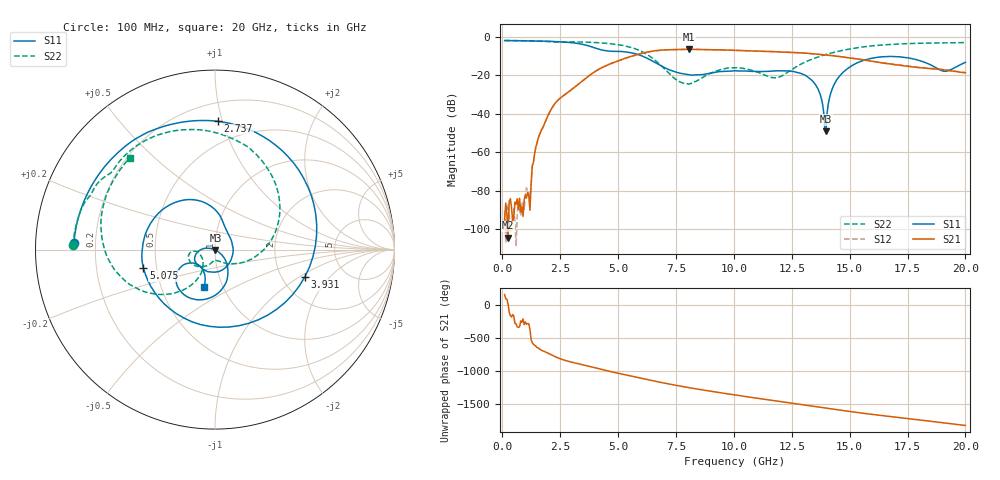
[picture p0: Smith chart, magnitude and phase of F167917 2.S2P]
!  2-Port S-parameters saved by WinCal
! VAR MeasName=S-Parameters (CALIBRATED_DATA) read from VNA (N5242A)
! VAR MeasDate=2016-11-22 8:59:41
! VAR NAME=F167917 2
! VAR FILENAME=F167917 2.S2P
! VAR DATE=2016-11-22 8:59:41
! VAR PHYS_PORTS=1,2
# Hz S DB R 50
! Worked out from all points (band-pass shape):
!   401 points, 100 MHz to 20 GHz, reference 50 ohm
!   highest |S21| = -6.61 dB at 8.06 GHz (marker M1); lowest = -104.4 dB at 249.2 MHz (marker M2)
!   |S21| within 3 dB of the highest: 5.744 GHz to 14.03 GHz (8.286 GHz wide, 83.8 % of centre)
!   lowest |S11| = -49.2 dB at 13.98 GHz (marker M3), VSWR 1.01, Z = 50.3 - j0.211 ohm
!   |S11| at or under -10 dB: 6.023 GHz to end of sweep
!   |S22| runs from -24.7 to -2.0 dB; largest |S21 - S12| = 0.0055
!   S11 on the Smith chart (normalised r, x): 100 MHz: 0.12, +0.02; 2.737 GHz: 0.33, +0.97; 3.931 GHz: 2.67, -1.11; 5.075 GHz: 0.42, -0.10; 20 GHz: 0.82, -0.35
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1e8  -2.09 177.3  -94.90 165.1  -90.39 46.4  -2.03 178.3
2.4925e8  -2.10 173.3  -104.37 19.3  -86.70 121.0  -2.04 175.9
1.14475e9  -2.25 149.1  -82.53 81.1  -80.87 95.1  -2.22 161.2
1.64225e9  -2.34 134.0  -49.88 48.9  -49.93 48.7  -2.44 153.8
2.73675e9  -2.92 88.6  -29.81 -118.6  -29.81 -118.9  -2.80 137.4
3.43325e9  -3.96 38.9  -23.27 -178.6  -23.29 -178.6  -2.83 123.3
3.93075e9  -5.63 -16.8  -18.73 138.7  -18.73 138.9  -3.05 111.2
4.42825e9  -7.27 -87.1  -15.40 95.1  -15.35 95.0  -3.45 97.2
5.075e9  -7.71 -165.6  -12.33 43.7  -12.29 43.2  -4.32 74.9
5.82125e9  -9.17 132.0  -9.35 -13.1  -9.36 -13.6  -6.69 39.7
6.7665e9  -14.61 80.5  -7.15 -84.8  -7.18 -84.9  -14.05 -17.4
8.06e9  -19.78 23.8  -6.61 -170.2  -6.63 -170.1  -24.67 -92.7
1.005e10  -17.74 -108.9  -7.15 78.1  -7.14 78.2  -16.21 -159.3
1.1841e10  -17.76 -140.3  -7.89 -13.2  -7.85 -13.1  -21.38 -148.2
1.338325e10  -22.92 177.6  -8.90 -92.0  -8.92 -91.8  -11.68 -125.7
1.368175e10  -28.50 167.6  -9.22 -107.1  -9.25 -106.8  -10.40 -129.9
1.398025e10  -49.23 -37.4  -9.59 -122.0  -9.57 -121.8  -9.29 -134.4
1.427875e10  -26.26 -37.8  -9.94 -137.1  -9.97 -136.6  -8.31 -139.4
1.47265e10  -18.45 -54.2  -10.60 -159.2  -10.59 -158.7  -7.09 -147.1
1.67165e10  -10.33 -120.5  -14.14 111.2  -14.07 111.5  -4.12 177.8
1.91045e10  -18.00 -133.2  -17.34 12.2  -17.20 12.2  -3.27 143.7
2e10  -13.36 -106.5  -18.82 -25.1  -18.64 -25.2  -3.14 132.7
